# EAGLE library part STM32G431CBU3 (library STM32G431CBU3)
MCU 32-bit ARM Cortex M4 RISC 128KB Flash 3.3V 48-Pin UFQFPN EP Tray Source: Datasheet
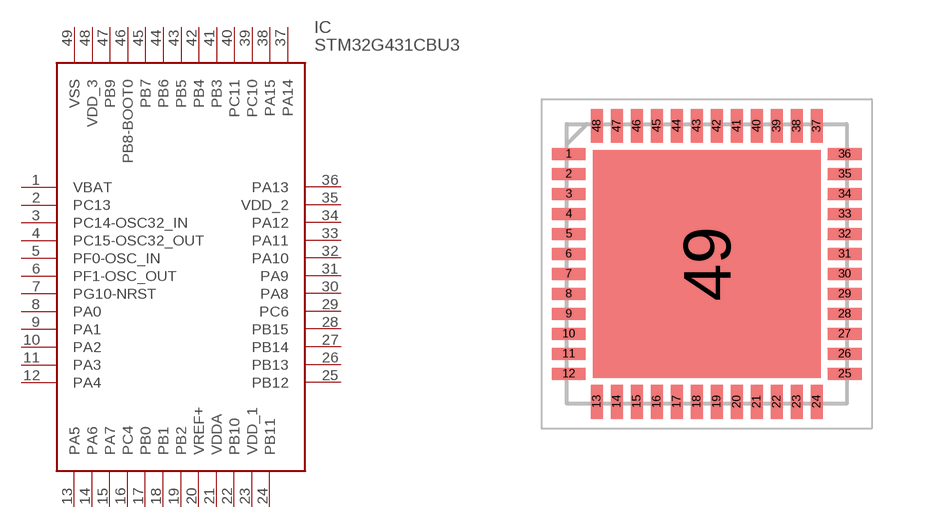
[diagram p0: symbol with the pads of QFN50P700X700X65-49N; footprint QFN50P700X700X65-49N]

Designator prefix IC

## STM32G431CBU3 (Description: MCU 32-bit ARM Cortex M4 RISC 128KB Flash 3.3V 48-Pin UFQFPN EP Tray; Height: 0.65mm; Manufacturer_Name: STMicroelectronics; Manufacturer_Part_Number: STM32G431CBU3; Mouser_Part_Number: 511-STM32G431CBU3; Mouser_Price-Stock: https://www.mouser.co.uk/ProductDetail/STMicroelectronics/STM32G431CBU3?qs=PzGy0jfpSMuhNWEWgwfZ0w%3D%3D)  [QFN50P700X700X65-49N]
1  VBAT
2  PC13
3  PC14-OSC32_IN
4  PC15-OSC32_OUT
5  PF0-OSC_IN
6  PF1-OSC_OUT
7  PG10-NRST
8  PA0
9  PA1
10  PA2
11  PA3
12  PA4
13  PA5
14  PA6
15  PA7
16  PC4
17  PB0
18  PB1
19  PB2
20  VREF+
21  VDDA
22  PB10
23  VDD_1
24  PB11
25  PB12
26  PB13
27  PB14
28  PB15
29  PC6
30  PA8
31  PA9
32  PA10
33  PA11
34  PA12
35  VDD_2
36  PA13
37  PA14
38  PA15
39  PC10
40  PC11
41  PB3
42  PB4
43  PB5
44  PB6
45  PB7
46  PB8-BOOT0
47  PB9
48  VDD_3
49  VSS

## Footprint QFN50P700X700X65-49N (pad centres in mm)
. UFQFPN48 - 48-lea
smd 0.85 x 0.3: 1 -3.45,2.75; 2 -3.45,2.25; 3 -3.45,1.75; 4 -3.45,1.25; 5 -3.45,0.75; 6 -3.45,0.25; 7 -3.45,-0.25; 8 -3.45,-0.75; 9 -3.45,-1.25; 10 -3.45,-1.75; 11 -3.45,-2.25; 12 -3.45,-2.75; 25 3.45,-2.75; 26 3.45,-2.25; 27 3.45,-1.75; 28 3.45,-1.25; 29 3.45,-0.75; 30 3.45,-0.25; 31 3.45,0.25; 32 3.45,0.75; 33 3.45,1.25; 34 3.45,1.75; 35 3.45,2.25; 36 3.45,2.75
smd 0.3 x 0.85: 13 -2.75,-3.45; 14 -2.25,-3.45; 15 -1.75,-3.45; 16 -1.25,-3.45; 17 -0.75,-3.45; 18 -0.25,-3.45; 19 0.25,-3.45; 20 0.75,-3.45; 21 1.25,-3.45; 22 1.75,-3.45; 23 2.25,-3.45; 24 2.75,-3.45; 37 2.75,3.45; 38 2.25,3.45; 39 1.75,3.45; 40 1.25,3.45; 41 0.75,3.45; 42 0.25,3.45; 43 -0.25,3.45; 44 -0.75,3.45; 45 -1.25,3.45; 46 -1.75,3.45; 47 -2.25,3.45; 48 -2.75,3.45
smd 5.7 x 5.7: 49 0,0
